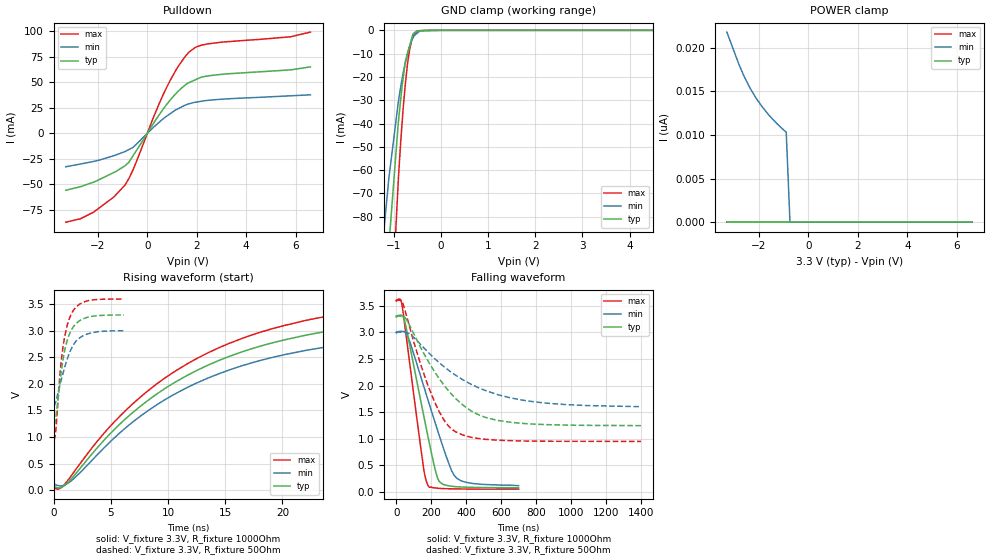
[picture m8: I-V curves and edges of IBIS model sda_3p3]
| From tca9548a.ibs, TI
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|   sda_3p3 Model
[Model]   sda_3p3
Model_type   I/O_open_drain
Polarity   Non-Inverting
Vinl  = 0.99
Vinh  =2.31
Vmeas = 1.65
Vref = 3.3
Cref = 50pF
Rref = 1000
|   typ   min   max
|   (nom PVT)   (fast PVT)   (slow PVT)
 C_comp   5.385e-12   4.670e-12   6.276e-12
[Model spec]
|subparameter
Vinl   0.99   0.9   1.08
Vinh   2.31   2.1   2.52
| Where nom  PVT is Nominal Process, 3.3V, 27C
|   Fast PVT is Strong Process,  3.6V, -40C
|   Slow PVT is Weak Process,   3V, 125C
[Voltage Range]   3.3   3   3.6
|Junction Temperature
[Temperature Range]   27   125   -40
[Pullup Reference]   3.3   3   3.6
[Pulldown Reference]   0   0   0
[Power Clamp Reference]   3.3   3   3.6
[GND Clamp Reference]   0   0   0
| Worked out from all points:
|   slope of the pulldown table from 0 to 0.495 V, typ, clamps not added: 26.6 ohm
|   GND clamp passes 1 mA (typ) near -0.56 V on its own axis
|   falling waveform, V_fixture 3.3V, R_fixture 1000Ohm: 20-80 % time 119ns typ, 167ns min, 84.8ns max; typ from 3.3 V to 0.08 V
|   rising waveform, V_fixture 3.3V, R_fixture 1000Ohm: 20-80 % time 13.7ns typ, 13.8ns min, 13.6ns max; typ from 0.08 V to 3.3 V
|   falling waveform, V_fixture 3.3V, R_fixture 50Ohm: 20-80 % time 260ns typ, 377ns min, 172ns max; typ from 3.3 V to 1.25 V
|   rising waveform, V_fixture 3.3V, R_fixture 50Ohm: 20-80 % time 937ps typ, 1.25ns min, 830ps max; typ from 1.25 V to 3.3 V
[Pulldown]
|   Voltage   I(typ)   I(min)   I(max)
-3.3V     -55.71mA   -32.76mA   -86.97mA
-2.182V   -47.88mA   -27.61mA   -77.22mA
-1.35V    -38.29mA   -21.85mA   -62.19mA
-896.4mV  -31.66mA   -17.79mA   -50.45mA
-568.8mV  -21.68mA   -13.54mA   -35.22mA
280.8mV   10.94mA    6.574mA    17.51mA
738mV     26.8mA     16.06mA    42.73mA
1.246V    41.05mA    24.06mA    65.31mA
1.706V    49.77mA    28.99mA    79.85mA
2.473V    56.17mA    32.3mA     87.59mA
5.8V      62.09mA    36.7mA     94.46mA
6.6V      65.02mA    37.66mA    99.04mA
[GND Clamp]
|   Voltage   I(typ)   I(min)   I(max)
-3.3V     -1.244A    -818.2mA   -1.716A
-1.318V   -166.7mA   -110.4mA   -254.8mA
-1.119V   -97.8mA    -67.79mA   -154.8mA
-1.098V   -92.33mA   -63.36mA   -144.3mA
-897.6mV  -39.39mA   -30.67mA   -63.94mA
-846mV    -29.32mA   -24.01mA   -47.44mA
-752.4mV  -13.85mA   -14.29mA   -23.59mA
-658.8mV  -6.681mA   -6.906mA   -8.292mA
-590.7mV  -1.734mA   -3.326mA   -2.954mA
-504.9mV  -361.2uA   -1.32mA    -487.1uA
-285mV    -202.8uA   -7.301uA   -2.542uA
6.6V      0A         0A         0A
[POWER Clamp]
|   Voltage   I(typ)   I(min)   I(max)
-3.3V     0A         21.78nA    0A
-2.802V   0A         18.01nA    0A
-2.592V   0A         16.64nA    0A
-2.367V   0A         15.39nA    0A
-2.124V   0A         14.24nA    0A
-1.863V   0A         13.19nA    0A
-1.575V   0A         12.19nA    0A
-896.4mV  0A         10.3nA     0A
-745.8mV  0A         0A         0A
6.6V      0A         0A         0A
[Ramp]
R_load = 1000
|   typ   min   max
dV/dt_r   1.93188/1.36667e-08   1.72837/1.37885e-08   2.12695/1.3648e-08
dV/dt_f   1.93177/1.18759e-07   1.72762/1.67142e-07   2.12694/8.47519e-08
[Falling Waveform]
V_fixture = 3.3V
V_fixture_min = 3V
V_fixture_max = 3.6V
R_fixture = 1000Ohm
|   Time   V(typ)   V(min)   V(max)
0s        3.3V       3V         3.6V
22.6ns    3.321V     3.017V     3.619V
32.4ns    3.315V     3.017V     3.519V
68ns      2.901V     2.901V     2.639V
158.2ns   1.413V     1.973V     402.9mV
186.2ns   964.1mV    1.677V     100.6mV
243.8ns   211mV      1.082V     71.02mV
316.2ns   110.2mV    403.5mV    61.25mV
345.8ns   100.9mV    261.1mV    59.58mV
699.8ns   80.37mV    120.6mV    55.09mV
[Rising Waveform]
V_fixture = 3.3V
V_fixture_min = 3V
V_fixture_max = 3.6V
R_fixture = 1000Ohm
|   Time   V(typ)   V(min)   V(max)
0s        80.18mV    119.3mV    55.07mV
600ps     43.03mV    77.93mV    33.71mV
1.4ns     173.1mV    150.3mV    226.3mV
5.8ns     1.244V     1.079V     1.393V
10.4ns    2.004V     1.787V     2.209V
15.4ns    2.523V     2.267V     2.769V
22ns      2.918V     2.631V     3.196V
28.4ns    3.119V     2.816V     3.409V
38.4ns    3.249V     2.949V     3.546V
69.32ns   3.3V       3V         3.6V
[Falling Waveform]
V_fixture = 3.3V
V_fixture_min = 3V
V_fixture_max = 3.6V
R_fixture = 50Ohm
|   Time   V(typ)   V(min)   V(max)
0s        3.3V       3V         3.6V
36.92ns   3.299V     3.001V     3.546V
139.7ns   2.712V     2.768V     2.393V
223.6ns   2.236V     2.493V     1.662V
282.1ns   1.968V     2.329V     1.308V
339.2ns   1.757V     2.193V     1.132V
467.7ns   1.455V     1.962V     1.007V
635.5ns   1.317V     1.782V     966.6mV
973.6ns   1.257V     1.641V     952.8mV
1.4us     1.248V     1.603V     951.6mV
[Rising Waveform]
V_fixture = 3.3V
V_fixture_min = 3V
V_fixture_max = 3.6V
R_fixture = 50Ohm
|   Time   V(typ)   V(min)   V(max)
0s        1.246V     1.594V     951.5mV
100ps     1.27V      1.607V     980.8mV
200ps     1.375V     1.67V      1.128V
540ps     1.991V     1.961V     2.131V
800ps     2.419V     2.177V     2.655V
1.14ns    2.779V     2.429V     3.057V
1.52ns    2.999V     2.649V     3.304V
2.1ns     3.164V     2.838V     3.476V
2.98ns    3.257V     2.944V     3.568V
6.16ns    3.301V     3.004V     3.601V
